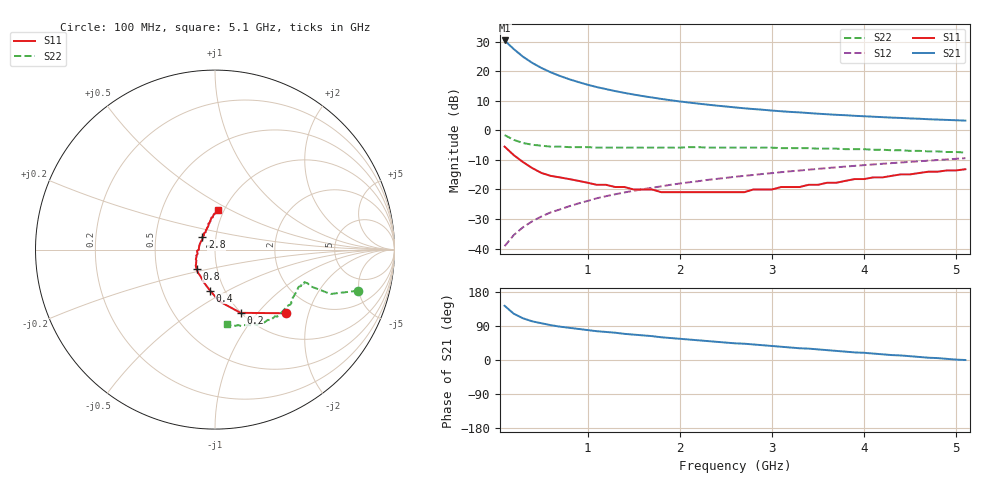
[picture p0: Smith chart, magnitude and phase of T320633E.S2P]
!AT-32063
!S AND NOISE PARAMETERS per side at Vce=2.7 V  Ic=20mA.  LAST UPDATED 11-11-96
# ghz s ma r 50
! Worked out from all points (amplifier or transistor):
!   51 points, 100 MHz to 5.1 GHz, reference 50 ohm
!   highest |S21| = 30.4 dB at 100 MHz (marker M1)
!   |S21| within 3 dB of that: start of sweep to 202.5 MHz
!   unconditionally stable (mu >= 1): 507.5 MHz to 3.976 GHz
!   at 900 MHz: K = 1.08, MAG = 18.8 dB, |S12| = -24.7 dB
!   at 2.6 GHz: K = 1.07, MAG = 10.1 dB, |S12| = -15.7 dB
!   at 5.1 GHz: K = 0.96, MSG = 6.4 dB, |S12| = -9.4 dB
!   lowest NFmin = 1.51 dB at 900 MHz
!   S11 on the Smith chart (normalised r, x): 100 MHz: 1.46, -1.44; 200 MHz: 1.00, -0.82; 400 MHz: 0.85, -0.41; 800 MHz: 0.80, -0.18; 2.8 GHz: 0.86, +0.12; 5.1 GHz: 0.94, +0.43
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0.1  0.53 -42.0  33.08 143.0  0.011 74.0  0.83 -16.0
0.2  0.38 -68.0  23.59 122.0  0.017 70.0  0.69 -21.0
0.3  0.29 -85.0  17.55 110.0  0.023 70.0  0.61 -21.0
0.4  0.23 -97.0  13.81 102.0  0.029 71.0  0.57 -21.0
0.5  0.19 -110.0  11.33 97.0  0.035 71.0  0.55 -20.0
0.6  0.17 -118.0  9.59 92.0  0.041 72.0  0.53 -20.0
0.7  0.16 -126.0  8.31 88.0  0.046 72.0  0.53 -21.0
0.8  0.15 -133.0  7.32 85.0  0.052 72.0  0.52 -21.0
0.9  0.14 -140.0  6.55 82.0  0.058 71.0  0.52 -22.0
1  0.13 -144.0  5.91 79.0  0.064 71.0  0.52 -23.0
1.1  0.12 -150.0  5.39 76.0  0.071 70.0  0.51 -24.0
1.2  0.12 -153.0  4.98 74.0  0.077 70.0  0.51 -24.0
1.4  0.11 -162.0  4.3 69.0  0.089 69.0  0.51 -26.0
1.6  0.1 -171.0  3.79 65.0  0.101 67.0  0.51 -29.0
1.8  0.09 -180.0  3.4 60.0  0.113 66.0  0.51 -31.0
2.2  0.09 162.0  2.83 52.0  0.138 62.0  0.52 -36.0
2.6  0.09 144.0  2.44 44.0  0.164 58.0  0.51 -41.0
2.8  0.1 135.0  2.29 41.0  0.176 56.0  0.51 -44.0
3.2  0.11 121.0  2.05 33.0  0.203 52.0  0.5 -49.0
3.5  0.12 113.0  1.91 28.0  0.223 49.0  0.49 -53.0
4.3  0.17 98.0  1.64 13.0  0.279 39.0  0.46 -66.0
5.1  0.22 86.0  1.46 0.0  0.338 30.0  0.42 -81.0
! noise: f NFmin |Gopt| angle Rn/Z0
0.9  1.51  0.13  88  0.2
1.8  1.78  0.2  178  0.13
2.4  1.96  0.28  -125  0.08
